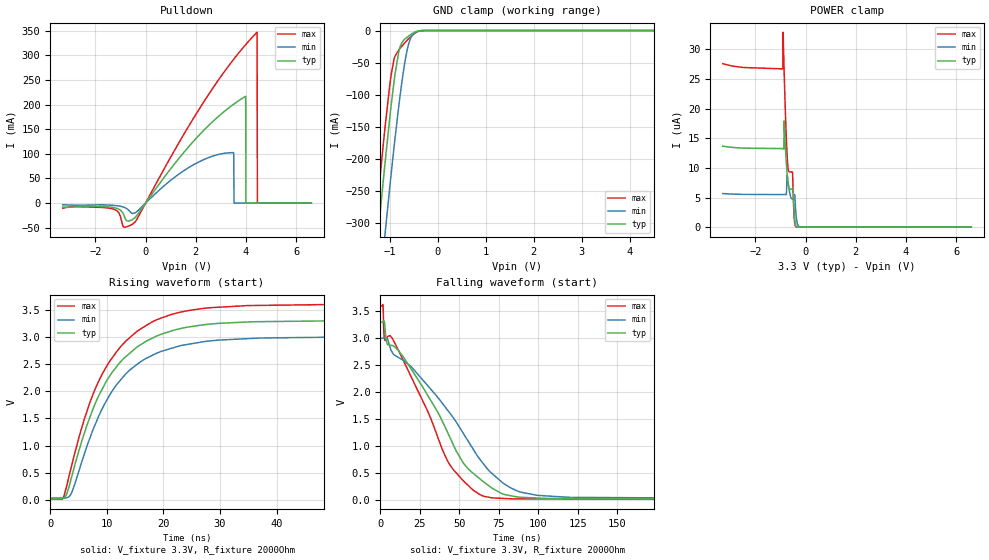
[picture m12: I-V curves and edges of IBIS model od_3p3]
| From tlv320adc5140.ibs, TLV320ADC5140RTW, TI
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|   od_3p3 Model
[Model]   od_3p3
Model_type   I/O_open_drain
Polarity   Non-Inverting
Enable   Active-Low
Vinl = 0.99
Vinh = 2.31
Vmeas = 1.65
Vref = 3.3
Cref = 2pF
Rref = 2000
|   typ   min   max
C_comp   1.666pF   1.613pF   1.721pF
[Model spec]
|subparameter
Vinl   0.99   0.9   1.08
Vinh   2.31   2.1   2.52
| Where Nom  PVT is Nominal Process, 3.3V, 27C
|   Fast PVT is Strong Process,  3.6V, -40C
|   Slow PVT is Weak Process,   3.0V, 150C
[Voltage Range]   3.3   3   3.6
|Junction Temperature
[Temperature Range]   27   150   -40
[Pullup Reference]   3.3   3   3.6
[Pulldown Reference]   0   0   -0
[Power Clamp Reference]   3.3   3   3.6
[GND Clamp Reference]   0   0   0
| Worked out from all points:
|   slope of the pulldown table from 0 to 0.495 V, typ, clamps not added: 14 ohm
|   GND clamp passes 1 mA (typ) near -0.42 V on its own axis
|   falling waveform, V_fixture 3.3V, R_fixture 2000Ohm: 20-80 % time 38ns typ, 45ns min, 32.8ns max; typ from 3.3 V to 0.024 V
|   rising waveform, V_fixture 3.3V, R_fixture 2000Ohm: 20-80 % time 8.97ns typ, 8.88ns min, 8.95ns max; typ from 0.024 V to 3.3 V
[Pulldown]
|   Voltage   I(typ)   I(min)   I(max)
-3.3V     -7.96mA    -3.343mA   -10.22mA
-1.29V    -8.797mA   -4.508mA   -11.75mA
-429mV    -29.86mA   -20.17mA   -38.81mA
1.66V     111.1mA    70.34mA    151.3mA
3.323V    193.7mA    102.1mA    279.6mA
3.511V    200.8mA    99.78mA    292.2mA
3.521V    201.2mA    145.7nA    292.8mA
3.986V    216.9mA    61.31nA    321.8mA
3.996V    2.432nA    61.06nA    322.3mA
4.442V    506.2pA    52.5nA     346.7mA
4.452V    504.3pA    52.35nA    10.86nA
6.6V      528.4pA    35.63nA    23.49pA
[GND Clamp]
|   Voltage   I(typ)   I(min)   I(max)
-3.3V     -2.029A    -2.056A    -2.018A
-1.31V    -368.6mA   -478.7mA   -312.1mA
-1.261V   -329.2mA   -439.6mA   -272.5mA
-1.221V   -298mA     -408.6mA   -241.3mA
-1.102V   -207.2mA   -317.6mA   -151.6mA
-973.5mV  -116.7mA   -223.5mA   -69.1mA
-914.1mV  -79.82mA   -182.3mA   -44.89mA
-815.1mV  -33.19mA   -118.2mA   -30.29mA
-636.9mV  -10.12mA   -29.47mA   -14.85mA
-557.7mV  -5.885mA   -10.48mA   -9.057mA
-458.7mV  -1.893mA   -2.535mA   -3.273mA
6.6V      0A         0A         0A
[POWER Clamp]
|   Voltage   I(typ)   I(min)   I(max)
-3.3V     13.66uA    5.669uA    27.59uA
-904.2mV  13.26uA    5.501uA    26.72uA
-894.3mV  13.26uA    5.501uA    32.89uA
-864.6mV  13.17uA    5.5uA      28.05uA
-854.7mV  17.94uA    5.5uA      26.5uA
-765.6mV  10.86uA    5.483uA    14.93uA
-716.1mV  8.125uA    8.287uA    10.82uA
-518.1mV  6.422uA    4.761uA    9.278uA
-458.7mV  3.167uA    5.072uA    1.965uA
-379.5mV  231.2nA    2.093uA    43.64nA
-122.1mV  0A         15.21nA    0A
6.6V      0A         0A         0A
[Ramp]
R_load = 2000
|   typ   min   max
dV/dt_r   1.96578/8.92962e-09   1.7802/8.87855e-09   2.1485/8.95082e-09
dV/dt_f   1.96578/3.80067e-08   1.7802/4.45868e-08   2.1485/3.27482e-08
[Falling Waveform]
V_fixture = 3.3V
V_fixture_min = 3V
V_fixture_max = 3.6V
R_fixture = 2000Ohm
C_fixture = 0F
|   Time   V(typ)   V(min)   V(max)
0s        3.3V       3V         3.6V
1.723ns   3.311V     3.005V     3.619V
2.779ns   3.274V     3.008V     2.97V
4.429ns   2.894V     2.999V     3.022V
9.833ns   2.823V     2.676V     2.878V
42.45ns   1.267V     1.675V     736.8mV
63.28ns   392mV      751.3mV    101.9mV
82.44ns   86.31mV    231.7mV    29.64mV
99.52ns   43.06mV    92.23mV    26.78mV
250ns     23.69mV    32.93mV    19.17mV
[Rising Waveform]
V_fixture = 3.3V
V_fixture_min = 3V
V_fixture_max = 3.6V
R_fixture = 2000Ohm
C_fixture = 0F
|   Time   V(typ)   V(min)   V(max)
0s        23.69mV    32.93mV    19.17mV
2.291ns   26.86mV    34.86mV    38.03mV
3.604ns   357.2mV    96.87mV    556.6mV
5.261ns   976.7mV    598.4mV    1.222V
7.508ns   1.663V     1.28V      1.935V
11.96ns   2.486V     2.151V     2.763V
17.95ns   2.976V     2.66V      3.277V
26.4ns    3.216V     2.903V     3.52V
49.38ns   3.298V     2.997V     3.598V
250ns     3.3V       3V         3.6V
